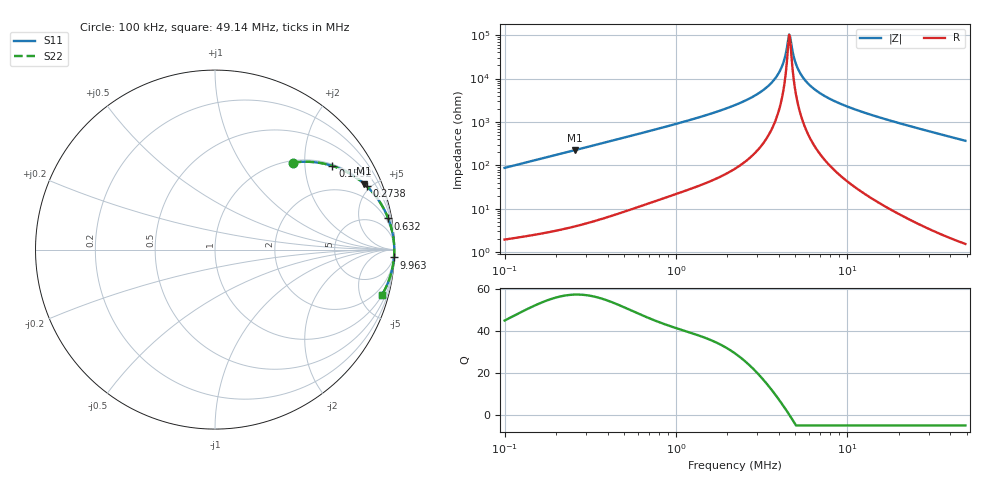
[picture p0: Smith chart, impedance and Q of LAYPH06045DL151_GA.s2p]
! LAYPH06045DL151_GA  S-PARAMETER MODEL  ( General Type )
! Model Generated by TAIYO YUDEN Corporation (http://www.ty-top.com)
! Version 2.0
! TAIYO YUDEN Control No. 180914NI43SB-FBB
! Copyright(c) 2018 TAIYO YUDEN CO.,LTD. All Rights Reserved.
! Product Description (link to TY-COMPAS)
! https://ds.yuden.co.jp/TYCOMPAS/or/detail?pn=LAYPH06045DL151MGA&u=M
! Products Name : Inductors
! Characteristics :
!  Inductance : 150 uH , SRF(min) : -Hz , DC Resistance(max) : 0.57 Ohm
!  Rated Current : Saturation :0.5 A , Temp Rise : 0.49 A (25 degC)
!  Case Size : 6.3 x 6.0 / 0.248 x 0.236 [mm/inch] , Thickness : 4.5 / 0.177 [mm/inch]
!  (Conditions: Temperature = 25 degC , DC Bias Current/Voltage = 0A / 0V)
! External Node Assignments :
!  1  o---GGG---o  2
! GND o---------o GND
! Frequency Range : 0.1MHz  -  49.142796MHz  [ 402 STEP ]
# MHz S RI R 50
! Freq[MHz].  S11 Real  S11 Imag  S21 Real  S21 Imag  S12 Real  S12 Imag  S22 Real  S22 Imag
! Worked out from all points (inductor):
!   401 points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, 100 kHz to 49.14 MHz, reference 50 ohm
!   read as one part in series: L = 139 uH near 103.1 kHz
!   highest Q = 57.3 at 257.3 kHz (marker M1), where L = 138 uH
!   self-resonance near 4.592 MHz
!   S11 on the Smith chart (normalised r, x): 100 kHz: 1.04, +1.75; 159.2 kHz: 1.05, +2.77; 273.8 kHz: 1.08, +4.76; 632 kHz: 1, +11; 9.963 MHz: 2, -46; 49.14 MHz: 1.03, -7.36
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0.1  0.434 0.4846  0.566 -0.4846  0.566 -0.4846  0.434 0.4846
0.159169  0.6546 0.4662  0.3454 -0.4662  0.3454 -0.4662  0.6546 0.4662
0.257305  0.8291 0.3678  0.1709 -0.3678  0.1709 -0.3678  0.8291 0.3678
0.273755  0.8456 0.3527  0.1544 -0.3527  0.1544 -0.3527  0.8456 0.3527
0.282371  0.8533 0.3451  0.1467 -0.3451  0.1467 -0.3451  0.8533 0.3451
0.631989  0.965 0.1735  0.035 -0.1735  0.035 -0.1735  0.965 0.1735
0.797332  0.9773 0.1381  0.0227 -0.1381  0.0227 -0.1381  0.9773 0.1381
2.251431  0.997 0.0397  0.00296 -0.0397  0.00296 -0.0397  0.997 0.0397
3.022059  0.9984 0.0222  0.00163 -0.0222  0.00163 -0.0222  0.9984 0.0222
3.696369  0.9988 0.0114  0.00116 -0.0114  0.00116 -0.0114  0.9988 0.0114
3.994097  0.999 0.00735  0.00105 -0.00735  0.00105 -0.00735  0.999 0.00735
4.184124  0.999 0.00496  0.001 -0.00496  0.001 -0.00496  0.999 0.00496
4.521139  0.999 0.000979  0.000952 -0.000979  0.000952 -0.000979  0.999 0.000979
4.591731  0.9991 0.000184  0.000946 -0.000184  0.000946 -0.000184  0.9991 0.000184
4.736241  0.9991 -0.0014  0.000939 0.0014  0.000939 0.0014  0.9991 -0.0014
4.961577  0.9991 -0.00379  0.000939 0.00379  0.000939 0.00379  0.9991 -0.00379
5.278789  0.999 -0.00699  0.000958 0.00699  0.000958 0.00699  0.999 -0.00699
6.259641  0.9989 -0.016  0.00113 0.016  0.00113 0.016  0.9989 -0.016
7.656352  0.9984 -0.0272  0.00159 0.0272  0.00159 0.0272  0.9984 -0.0272
9.963432  0.9973 -0.0435  0.00273 0.0435  0.00273 0.0435  0.9973 -0.0435
17.67539  0.9908 -0.091  0.0092 0.091  0.0092 0.091  0.9908 -0.091
49.1428  0.9303 -0.2526  0.0697 0.2526  0.0697 0.2526  0.9303 -0.2526
